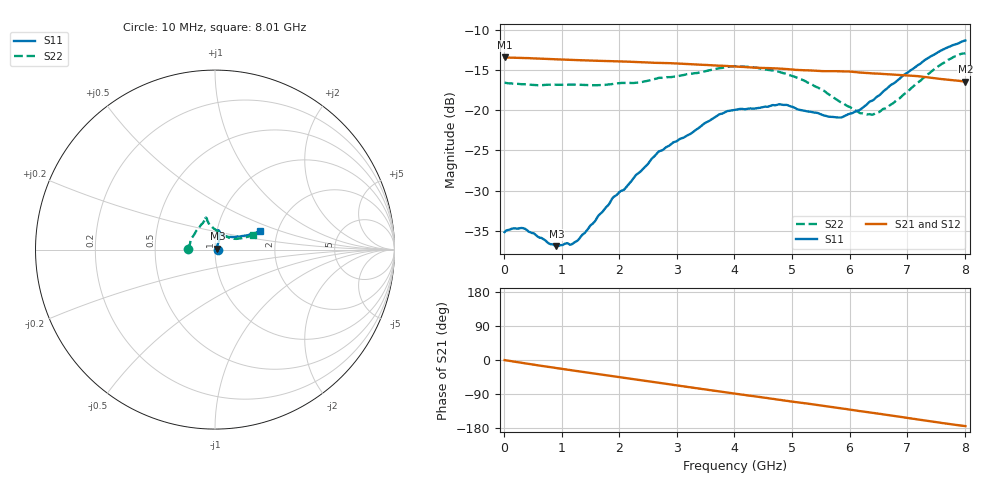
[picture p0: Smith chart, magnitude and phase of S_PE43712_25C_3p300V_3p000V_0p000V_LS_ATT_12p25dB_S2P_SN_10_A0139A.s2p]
! DEVICE ID: PE43712
! File Path: z:\PE43713\PE43713_CHAR_NOM_04292014\AMB\3p300\LS_ATT_12p25dB\PE43713_AMB_3p300V_3p000V_0p000V_LS_ATT_12p25dB_S2P_SN_10_A0139A.s2p
! Serial: 10
! Lot: A0139A
! Temp: 25C
! VDD: 3.300
! VSS: 0.000
! Control_Hi: 3.000
! Control_Lo: 0.000
! Attenuation Step: 12.25dB
! Port 1: RF1
! Port 2: RF2
! ThroughPath:1-2
! IDD: 0.0001469908
! ISS: -9.22e-008
#  Hz  S  RI  R  50
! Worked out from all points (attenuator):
!   801 points, 10 MHz to 8.01 GHz, reference 50 ohm
!   highest |S21| = -13.45 dB at 10 MHz (marker M1); lowest = -16.5 dB at 8.01 GHz (marker M2)
!   lowest |S11| = -36.9 dB at 910 MHz (marker M3), VSWR 1.03, Z = 51.3 + j0.52 ohm
!   |S11| at or under -10 dB: start of sweep to end of sweep
!   |S22| runs from -20.6 to -12.9 dB; largest |S21 - S12| = 0.00079
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1e7  0.0174 0.000288  0.2126 -0.00112  0.2128 -0.00105  -0.1481 0.001
1.6e8  0.0184 0.00063  0.2115 -0.0148  0.2116 -0.0147  -0.1459 0.0101
3.4e8  0.0184 0.000325  0.2085 -0.0305  0.2085 -0.03  -0.1437 0.0186
9.1e8  0.0133 0.00507  0.1929 -0.0756  0.193 -0.0756  -0.1359 0.0473
1.18e9  0.0114 0.00932  0.1823 -0.0941  0.1823 -0.0942  -0.1307 0.0611
1.35e9  0.0115 0.012  0.1752 -0.1052  0.1752 -0.1052  -0.1264 0.0684
1.9e9  0.0135 0.0254  0.1475 -0.1373  0.1475 -0.1373  -0.1091 0.097
2.1e9  0.0144 0.0292  0.1359 -0.1474  0.136 -0.1473  -0.1036 0.105
2.68e9  0.0228 0.0501  0.0986 -0.1701  0.0986 -0.1701  -0.0778 0.1382
3.72e9  0.0233 0.0903  0.0247 -0.1876  0.0246 -0.1876  -0.0549 0.1731
4.01e9  0.0219 0.0982  0.00412 -0.187  0.00411 -0.187  -0.055 0.1796
4.79e9  0.0197 0.1071  -0.0475 -0.1748  -0.0475 -0.1749  -0.0451 0.1665
5.35e9  0.0303 0.0923  -0.0795 -0.1574  -0.0795 -0.1573  -0.0323 0.1407
5.64e9  0.0407 0.0815  -0.0943 -0.1473  -0.0942 -0.1474  -0.0146 0.1246
5.88e9  0.0516 0.0746  -0.1074 -0.1373  -0.1072 -0.1373  0.00349 0.1108
6.17e9  0.0706 0.071  -0.1205 -0.122  -0.1203 -0.1221  0.0304 0.0914
6.3e9  0.083 0.0701  -0.1251 -0.1154  -0.1249 -0.1153  0.0441 0.083
6.42e9  0.0928 0.07  -0.1293 -0.1092  -0.1291 -0.1092  0.0562 0.0759
6.68e9  0.1204 0.0712  -0.1377 -0.0945  -0.1375 -0.0945  0.0841 0.0645
7.55e9  0.2136 0.0883  -0.1516 -0.0401  -0.1514 -0.0402  0.1752 0.0696
7.81e9  0.2355 0.0981  -0.1514 -0.0254  -0.1514 -0.0255  0.1997 0.0785
8.01e9  0.25 0.1054  -0.1496 -0.0147  -0.1494 -0.0149  0.2104 0.0818
